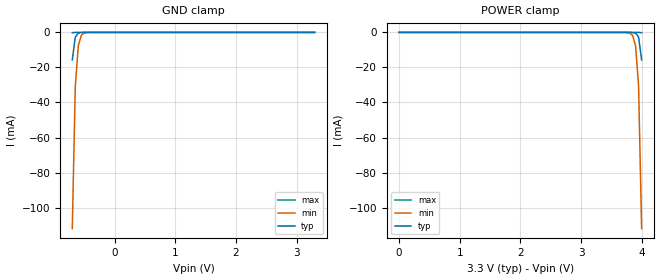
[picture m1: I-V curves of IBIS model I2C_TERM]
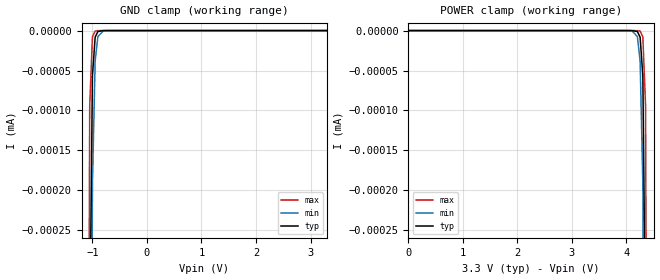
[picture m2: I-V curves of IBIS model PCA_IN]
|   NXP Semiconductors Inc.
|   Specialty Logic Products Group
|   IBIS model of PCA9546A
|   4-Channel I2C switch with reset
[IBIS Ver]   3.2
[Comment Char]   |_char
| VDD TYP:3.3V, MIN:2.97V, MAX: 3.63V
[File name]   pca9546a_3_3v.ibs
[File Rev]   1.0
[Date]   Dec 14, 2007 10:28:50 AM
[Source]
Generated by Seshadri Venkataramanan with IbisToolKit at Tempe, AZ
[Notes]
[Disclaimer]
(C) Copyright 2007 NXP Semiconductors
All rights reserved
NXP Semiconductors (NXP) does not warrant that this model and any other
accompanying information (Model) accurately or fully represents the
operating characteristics and specifications of the semiconductor
products to which the Model relates.  Moreover, the Model is furnished
on an "as is" and with "all faults" basis, and without support or
warranty of any kind.  NXP disclaims all warranties, whether expressed
or implied or statutory, including without limitation all implied
warranties of non-infringement, merchantability and fitness for any
purpose, and those arising from a course of dealing or usage of trade.
NXP does not convey any license under its or any third party's patents,
copyrights or other intellectual property or proprietary rights.
You and your company assume any and all risks and liability arising out
of the application or use of the Model.
In no event shall NXP be liable for any direct, indirect, special,
consequential or incidental damages, however caused, whether in
warranty, contract or tort (including negligence), strict liability or
other legal theory, including, without limitation, for lost profits,
business interruption, or corruption or loss of data or information,
arising out of or in connection with the use of or the inability to use
the Model, even if NXP has been advised of the possibility of such
damages.
NXP provides the Model as a courtesy to our customers. You and your
company shall not distribute, convey, sell, or give the Model to anyone
else without receiving prior written permission from NXP.
NXP reserves the right to make changes without notice to the Model to
improve reliability, function, or design.
Please be aware that your receipt and subsequent use of the Model shall
serve as acceptance of these terms and conditions.  If you do not
accept these terms, return or destroy the Model immediately.
[Copyright]
2007
[Component]   PCA9546AD
Si_location Pin
Timing_location Pin
[Manufacturer]   NXP Semiconductors
[Package]
|   variable   typ   min   max
R_pkg   1.75E-01   1.28E-01   2.11E-01
L_pkg   5.03E-09   3.94E-09   6.26E-09
C_pkg   0.794E-12   0.715E-12   0.869E-12
|  SO16
[Pin] signal_name   model_name   R_pin   L_pin   C_pin
1   A0   PCA_IN   1.99E-01  6.26E-09  0.822E-12
2   A1   PCA_IN   2.11E-01  5.46E-09  0.869E-12
3   RESETB   PCA_IN   1.56E-01  4.44E-09  0.760E-12
4   SD0   I2C_TERM   1.28E-01  3.94E-09  0.717E-12
5   SC0   I2C_TERM   1.28E-01  3.94E-09  0.715E-12
6   SD1   I2C_TERM   1.56E-01  4.44E-09  0.760E-12
7   SC1   I2C_TERM   2.11E-01  5.46E-09  0.869E-12
8   Vss   GND   1.99E-01  6.26E-09  0.843E-12
9   SD2   I2C_TERM   1.99E-01  6.26E-09  0.843E-12
10   SC2   I2C_TERM   2.11E-01  5.46E-09  0.869E-12
11   SD3   I2C_TERM   1.56E-01  4.44E-09  0.760E-12
12   SC3   I2C_TERM   1.28E-01  3.94E-09  0.717E-12
13   A2   PCA_IN   1.28E-01  3.94E-09  0.715E-12
14   SCL   I2C_TERM   1.56E-01  4.44E-09  0.760E-12
15   SDA   I2C_TERM   2.11E-01  5.46E-09  0.869E-12
16   Vdd   POWER   1.99E-01  6.26E-09  0.843E-12
[Series Pin Mapping] pin_2 model_name   function_table_group
14   5   PCA_SW   1
14   7   PCA_SW   2
14   10   PCA_SW   3
14   12   PCA_SW   4
15   6   PCA_SW   2
15   4   PCA_SW   1
15   11   PCA_SW   4
15   9   PCA_SW   3
[Series Switch Groups]
Off 1 2 3 4 /
On 1 /
On 2 /
On 3 /
On 4 /
[Component]   PCA9546APW
Si_location Pin
Timing_location Pin
[Manufacturer]   NXP Semiconductors
[Package]
|   variable   typ   min   max
R_pkg   3.44E-02   2.80E-02   4.33E-02
L_pkg   1.83E-09   1.36E-09   2.32E-09
C_pkg   0.380E-12   0.302E-12   0.442E-12
|  TSSOP16
[Pin] signal_name   model_name   R_pin   L_pin   C_pin
1   A0   PCA_IN   3.52E-02  2.40E-09  0.436E-12
2   A1   PCA_IN   3.70E-02  1.93E-09  0.438E-12
3   RESETB   PCA_IN   4.56E-02  1.76E-09  0.345E-12
4   SD0   I2C_TERM   4.00E-02  1.65E-09  0.335E-12
5   SC0   I2C_TERM   4.00E-02  1.65E-09  0.335E-12
6   SD1   I2C_TERM   4.56E-02  1.76E-09  0.345E-12
7   SC1   I2C_TERM   3.70E-02  1.93E-09  0.438E-12
8   Vss   GND   3.52E-02  2.40E-09  0.452E-12
9   SD2   I2C_TERM   3.52E-02  2.40E-09  0.452E-12
10   SC2   I2C_TERM   3.70E-02  1.93E-09  0.438E-12
11   SD3   I2C_TERM   4.56E-02  1.76E-09  0.345E-12
12   SC3   I2C_TERM   4.00E-02  1.65E-09  0.771E-12
13   A2   PCA_IN   4.00E-02  1.65E-09  0.771E-12
14   SCL   I2C_TERM   4.56E-02  1.76E-09  0.345E-12
15   SDA   I2C_TERM   3.70E-02  1.93E-09  0.438E-12
16   Vdd   POWER   3.52E-02  2.40E-09  0.452E-12
[Series Pin Mapping] pin_2 model_name   function_table_group
14   5   PCA_SW   1
14   7   PCA_SW   2
14   10   PCA_SW   3
14   12   PCA_SW   4
15   4   PCA_SW   1
15   6   PCA_SW   2
15   9   PCA_SW   3
15   11   PCA_SW   4
[Series Switch Groups]
Off 1 2 3 4 /
On 1 /
On 2 /
On 3 /
On 4 /
[Component]   PCA9546ABS
Si_location Pin
Timing_location Pin
[Manufacturer]   NXP Semiconductors
[Package]
|   [Package]   HVQFN16 (uses tssop24 data here only)
|   variable   typ   min   max
R_pkg   3.44E-02   2.80E-02   4.33E-02
L_pkg   1.83E-09   1.36E-09   2.32E-09
C_pkg   0.380E-12   0.302E-12   0.442E-12
|  HVQFN16
[Package Model]   hvqfn16
[Pin] signal_name   model_name
1   RESETB   PCA_IN
2   SD0   I2C_TERM
3   SC0   I2C_TERM
4   SD1   I2C_TERM
5   SC1   I2C_TERM
6   Vss   GND
7   SD2   I2C_TERM
8   SC2   I2C_TERM
9   SD3   I2C_TERM
10   SC3   I2C_TERM
11   A2   I2C_TERM
12   SCL   I2C_TERM
13   SDA   I2C_TERM
14   Vdd   POWER
15   A0   PCA_IN
16   A1   PCA_IN
[Series Pin Mapping] pin_2 model_name   function_table_group
12   3   PCA_SW   1
12   5   PCA_SW   2
12   8   PCA_SW   3
12   10   PCA_SW   4
13   2   PCA_SW   1
13   4   PCA_SW   2
13   7   PCA_SW   3
13   9   PCA_SW   4
[Series Switch Groups]
|   Function Group States
| default
Off 1 2 3 4 /
On 1 /
On 2 /
On 3 /
On 4 /
| [End   I2C_TERM
[Define Package Model]   hvqfn16
[Manufacturer]   Unknown
[OEM]   Unknown
[Description]   For pca9544a and pca9545a
[Number of Pins]   16
[Pin Numbers]
|   1 = D2
1
|   2 = D3
2
|   3 = D4
3
|   4 = D5
4
|   5 = D6
5
|   6 = D7
6
|   7 = NC
7
|   8 = Vss
8
|   9 = WRn
9
|   10 = RDn
10
|   11 = CEn
11
|   12 = A0
12
|   13 = A1
13
|   14 = INTn
14
|   15 = RESETn
15
|   16 = SCL
16
|   17 = SDA
|   18 = Vdd
|   19 = D0
|   20 = D1
[Model Data]
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[End Model Data]
[End Package Model]
[Model]   PCA_SW
Model_type Series_switch
C_comp   2.51p   2.51p   2.51p
[Temperature Range] 27   85   -40
[Voltage Range]   3.3   2.97   3.63
[Pullup Reference]  3.3   2.97   3.63
[Pulldown Reference]0   0   0
[On]
[R Series]   9   4   24
[L Series]   1n   1n   1n
[C Series]   1p   1p   1p
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[Off]
|   variable   R(typ)   R(min)   R(max)
[R Series]   1e06   1e06   1e06
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| Models and submodels in the file (3): I2C_TERM (Terminator), PCA_IN (Input), PCA_SW (Series_switch)
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[Model]   I2C_TERM
Model_type Terminator
C_comp   9.5p   9.5p   9.5p
[Temperature Range] 27   85   -40
[Voltage Range]   3.3   2.97   3.63
[Pullup Reference]  3.3   2.97   3.63
[Pulldown Reference]0   0   0
[POWER Clamp Reference]3.3   2.97   3.63
[GND Clamp Reference]0   0   0
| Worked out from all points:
|   GND clamp passes 1 mA (typ) near -0.61 V on its own axis
[GND Clamp]
|   -6.000000E-1   -1.554225E-1   -1.242642E-1   -2.666059E-1
|   -5.000000E-1   -1.602113E-1   -1.179351E-1   -2.662641E-1
|   -4.000000E-1   -1.574088E-1   -1.099432E-1   -2.800035E-1
-700mV    -15.71mA   -112mA     -166.1uA
-650mV    -2.644mA   -30.67mA   -13.81uA
-600mV    -395.5uA   -7.558mA   -1.147uA
-550mV    -57.52uA   -1.64mA    -95.33nA
-500mV    -8.329uA   -332.4uA   -8.003nA
-400mV    -174.5nA   -13.1uA    -133.3pA
3.3V      580.2pA    638.9pA    606.2pA
[POWER Clamp]
0V        580.2pA    638.9pA    606.2pA
3.7V      -174.5nA   -13.1uA    -133.3pA
3.8V      -8.329uA   -332.4uA   -8.003nA
3.85V     -57.52uA   -1.64mA    -95.33nA
3.9V      -395.5uA   -7.558mA   -1.147uA
3.95V     -2.644mA   -30.67mA   -13.81uA
4V        -15.71mA   -112mA     -166.1uA
[Model]   PCA_IN
Model_type Input
Vinh=2.1
Vinl=0.9
C_comp   1.73p   1.73p   1.73p
[Temperature Range] 27   85   -40
[Voltage Range]   3.3   2.97   3.63
[POWER Clamp Reference]3.3   2.97   3.63
[GND Clamp Reference]0   0   0
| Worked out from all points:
|   GND clamp passes 1 mA (typ) near -1.25 V on its own axis
[GND Clamp]
-2V       -10.17A    -9.093A    -11.52A
-1.1V     -2.718uA   -4.916uA   -1.14uA
-1.05V    -393.3nA   -972.8nA   -94.64nA
-1V       -56.9nA    -192.5nA   -7.858nA
-950mV    -8.234nA   -38.09nA   -653.2pA
-900mV    -1.192nA   -7.538nA   -55.05pA
-800mV    -25.74pA   -295.9pA   -1.173pA
3.3V      3.3pA      3.3pA      3.3pA
[POWER Clamp]
0V        3.3pA      3.3pA      3.3pA
4.1V      -25.74pA   -296pA     -1.173pA
4.2V      -1.192nA   -7.539nA   -55.05pA
4.25V     -8.234nA   -38.1nA    -653.2pA
4.3V      -56.9nA    -192.5nA   -7.858nA
4.35V     -393.3nA   -973nA     -94.64nA
4.4V      -2.718uA   -4.917uA   -1.14uA
5.3V      -10.17A    -9.093A    -11.52A
